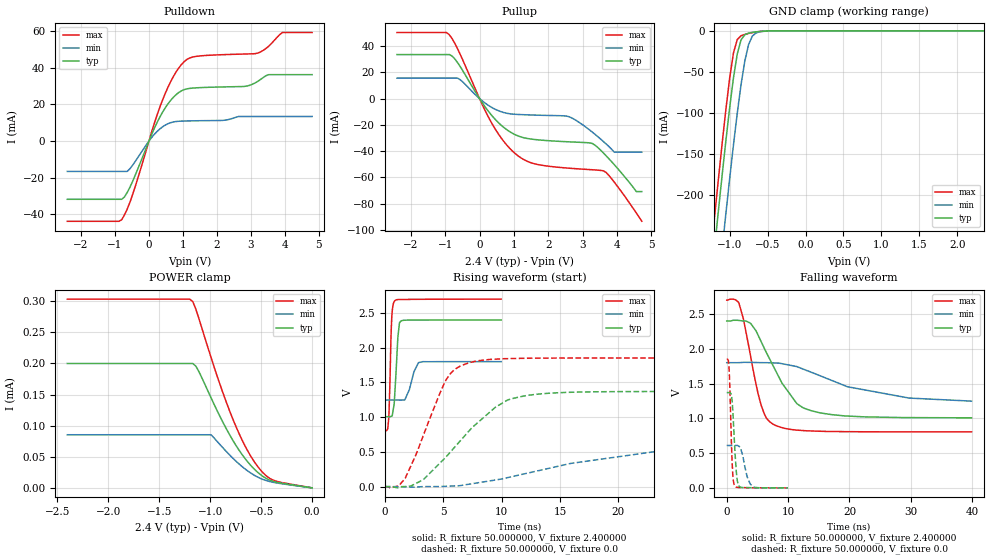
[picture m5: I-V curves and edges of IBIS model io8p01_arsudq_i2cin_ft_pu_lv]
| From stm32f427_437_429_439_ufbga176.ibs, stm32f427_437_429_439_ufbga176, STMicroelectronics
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|   Model io8p01_arsudq_i2cin_ft_pu_lv
[Model]  io8p01_arsudq_i2cin_ft_pu_lv
Model_type I/O
Polarity   Non-Inverting
Enable   Active-Low
Vinl =   0.720000V
Vinh =   1.680000V
Vmeas =  1.200000V
Cref =   50.000000pF
Rref =   100.000000M
Vref =   0.0V
C_comp   2.230300pF   2.174000pF   2.332300pF
[Temperature Range]   25.000000   0.125000k   -40.000000
[Pullup Reference]   2.400000V   1.800000V   2.700000V
[Pulldown Reference]   0.0V   0.0V   0.0V
[POWER Clamp Reference]   2.400000V   1.800000V   2.700000V
[GND Clamp Reference]   0.0V   0.0V   0.0V
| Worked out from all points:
|   slope of the pulldown table from 0 to 0.36 V, typ, clamps not added: 25 ohm
|   slope of the pullup table from 0 to 0.36 V, typ, clamps not added: 27.7 ohm
|   GND clamp passes 1 mA (typ) near -0.62 V on its own axis
|   rising waveform, R_fixture 50.000000, V_fixture 2.400000: 20-80 % time 273ps typ, 604ps min, 184ps max; typ from 1.01 V to 2.4 V
|   rising waveform, R_fixture 50.000000, V_fixture 0.0: 20-80 % time 4.82ns typ, 12.1ns min, 2.65ns max; typ from 0.001 V to 1.37 V
|   falling waveform, R_fixture 50.000000, V_fixture 2.400000: 20-80 % time 5.3ns typ, 12.6ns min, 2.67ns max; typ from 2.4 V to 1.01 V
|   falling waveform, R_fixture 50.000000, V_fixture 0.0: 20-80 % time 525ps typ, 974ps min, 385ps max; typ from 1.37 V to 0.001 V
[Pulldown]
|Voltage   I(typ)   I(min)   I(max)
-2.4V     -31.73mA   -16.51mA   -43.74mA
-800mV    -31.73mA   -16.51mA   -42.87mA
-480mV    -21.98mA   -13.17mA   -29.21mA
80mV      3.63mA     1.966mA    5.014mA
480mV     18.16mA    8.738mA    26.02mA
800mV     25.38mA    10.72mA    37.77mA
1.12V     28.53mA    11.02mA    44.6mA
2.8V      29.84mA    13.46mA    47.53mA
3.2V      32.6mA     13.46mA    48.03mA
3.52V     36.28mA    13.46mA    51.75mA
3.92V     36.28mA    13.46mA    59.24mA
4.8V      36.28mA    13.46mA    59.24mA
[Pullup]
|Voltage   I(typ)   I(min)   I(max)
-2.4V     33.5mA     15.55mA    50.22mA
-960mV    33.5mA     15.55mA    50.22mA
-560mV    24.27mA    14.29mA    33.52mA
320mV     -11.75mA   -6.207mA   -17.08mA
960mV     -26.47mA   -11.82mA   -40.02mA
1.52V     -30.88mA   -12.51mA   -49.05mA
2.56V     -32.88mA   -13.48mA   -52.9mA
3.28V     -34.18mA   -25.52mA   -54.17mA
3.6V      -41.3mA    -32.61mA   -54.97mA
3.92V     -50.32mA   -40.8mA    -63.62mA
4.56V     -70.8mA    -40.8mA    -87.07mA
4.72V     -70.8mA    -40.8mA    -93.4mA
[GND_clamp]
|Voltage   I(typ)   I(min)   I(max)
-2.4V     -1.424A    -1.508A    -1.393A
-1.25V    -311.2mA   -401.9mA   -273.3mA
-1.2V     -265.4mA   -356.1mA   -227.2mA
-1.15V    -220.4mA   -310.8mA   -181.9mA
-1.1V     -176.3mA   -266.2mA   -137.9mA
-1.05V    -133.8mA   -222.5mA   -95.87mA
-950mV    -57.3mA    -138.9mA   -26.98mA
-900mV    -28.27mA   -100.4mA   -10.59mA
-850mV    -11.01mA   -65.54mA   -5.958mA
-750mV    -2.834mA   -16.5mA    -3.178mA
-600mV    -750uA     -1.164mA   -738.3uA
2.35V     0A         0A         0A
[POWER_clamp]
|Voltage   I(typ)   I(min)   I(max)
-2.4V     200uA      85.39uA    303.5uA
-1.2V     200uA      85.39uA    303.5uA
-1.17V    200uA      85.39uA    299.5uA
-1.14V    195.7uA    85.39uA    287.5uA
-990mV    144.6uA    85.39uA    209.3uA
-870mV    104.1uA    63.61uA    150.8uA
-780mV    77.28uA    48.2uA     111.8uA
-660mV    47.71uA    30.75uA    68.21uA
-570mV    30.64uA    20.61uA    42.79uA
-480mV    18.19uA    13.44uA    24.07uA
-390mV    10.91uA    9.231uA    13.01uA
0V        0A         0A         0A
[Ramp]
| variable   typ   min   max
dV/dt_r  0.82207/4.81262n   0.38468/13.01116n   1.11083/2.64539n
dV/dt_f  0.83592/5.30439n   0.32280/13.33949n   1.13691/2.66828n
R_load = 50.000000
[Rising Waveform]
R_fixture= 50.000000
V_fixture= 2.400000
V_fixture_min= 1.800000
V_fixture_max= 2.700000
|time   V(typ)   V(min)   V(max)
0s        1.007V     1.247V     805.7mV
240.2ps   1.007V     1.247V     826.6mV
340.3ps   1.007V     1.247V     989.3mV
600.6ps   1.016V     1.247V     2.444V
860.9ps   1.349V     1.247V     2.678V
1.121ns   2.15V      1.247V     2.693V
1.381ns   2.384V     1.246V     2.694V
1.722ns   2.396V     1.253V     2.695V
2.903ns   2.398V     1.786V     2.697V
9.97ns    2.4V       1.8V       2.7V
[Rising Waveform]
R_fixture= 50.000000
V_fixture= 0.0
V_fixture_min= 0.0
V_fixture_max= 0.0
|time   V(typ)   V(min)   V(max)
0s        1.058mV    913.7uV    1.345mV
1.201ns   -11.86mV   972.2uV    12.66mV
1.762ns   1.865mV    233uV      125.9mV
3.283ns   100.7mV    1.332mV    729.3mV
5.125ns   406.9mV    5.331mV    1.5V
7.287ns   815.9mV    37.92mV    1.786V
10.49ns   1.245V     129.7mV    1.843V
13.21ns   1.334V     232.6mV    1.85V
24.82ns   1.37V      544.5mV    1.853V
39.88ns   1.371V     610.2mV    1.853V
[Falling Waveform]
R_fixture= 50.000000
V_fixture= 2.400000
V_fixture_min= 1.800000
V_fixture_max= 2.700000
|time   V(typ)   V(min)   V(max)
0s        2.4V       1.8V       2.7V
2.002ns   2.407V     1.801V     2.653V
3.924ns   2.362V     1.805V     1.876V
5.606ns   2.104V     1.801V     1.189V
7.688ns   1.734V     1.796V     909.6mV
11.37ns   1.218V     1.745V     831.4mV
13.77ns   1.11V      1.662V     818.8mV
19.7ns    1.033V     1.454V     808.9mV
29.71ns   1.011V     1.292V     806.1mV
39.88ns   1.007V     1.247V     805.7mV
[Falling Waveform]
R_fixture= 50.000000
V_fixture= 0.0
V_fixture_min= 0.0
V_fixture_max= 0.0
|time   V(typ)   V(min)   V(max)
0s        1.371V     610.2mV    1.853V
380.4ps   1.371V     610.2mV    1.718V
480.5ps   1.371V     610.2mV    1.521V
880.9ps   1.254V     610mV      368.3mV
1.041ns   1.034V     609.7mV    134mV
1.261ns   650.4mV    609.6mV    37.79mV
1.702ns   118.8mV    611.6mV    8.3mV
2.062ns   20.22mV    593.9mV    6.304mV
3.864ns   3.608mV    52.4mV     2.581mV
9.97ns    1.058mV    913.7uV    1.345mV
